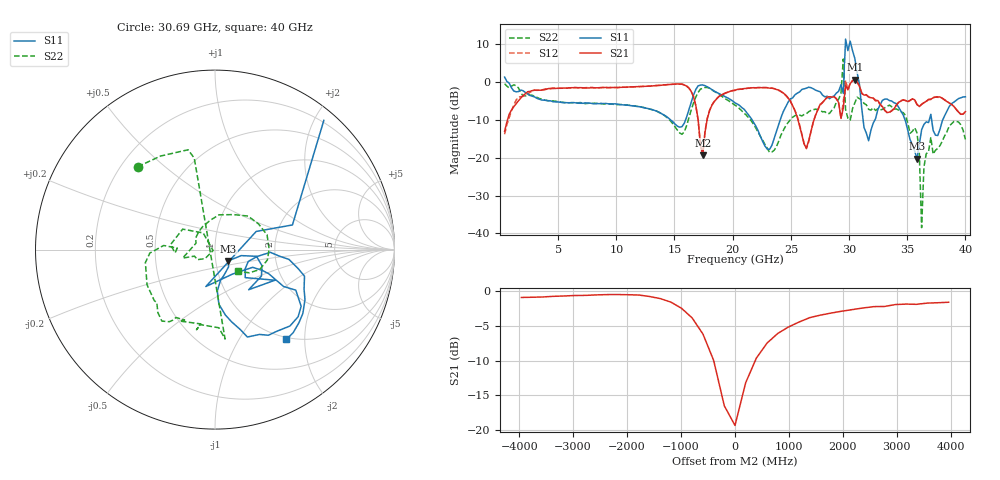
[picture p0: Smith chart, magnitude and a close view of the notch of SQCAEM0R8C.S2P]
! Network Analyzer HP8722ES.07.66: Jul 25, 2000 Serial No. US39175408
! 26 Oct 2004  09:32:31
! Frequency  S11  S21  S12  S22
# HZ  S  DB R  50
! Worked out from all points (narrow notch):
!   201 points, 400 MHz to 40 GHz, reference 50 ohm
!   highest |S21| = 0.61 dB at 30.5 GHz (marker M1); lowest = -19.3 dB at 17.43 GHz (marker M2)
!   notch at M2: 16.8 dB deep, 691 MHz wide at half that depth
!   lowest |S11| = -20.3 dB at 35.84 GHz (marker M3), VSWR 1.21, Z = 57.5 - j7.3 ohm
!   |S11| at or under -10 dB: 14.66 GHz to 15.95 GHz (1.287 GHz wide, 8.41 % of centre); 21.67 GHz to 24.09 GHz (2.415 GHz wide, 10.6 % of centre); 34.81 GHz to 36.9 GHz (2.081 GHz wide, 5.8 % of centre)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
!   |S22| runs from -38.5 to 6.1 dB; largest |S21 - S12| = 0.26
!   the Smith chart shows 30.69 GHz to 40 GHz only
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4e8  1.31 -10.9  -13.01 79.4  -13.79 83.7  -0.44 -5.1
7.132e9  -5.60 -84.4  -1.52 -7.7  -1.53 -8.7  -5.62 -113.3
1.3666e10  -7.94 -83.6  -0.87 -37.5  -0.85 -38.1  -8.04 -172.0
1.6042e10  -9.26 -21.5  -1.07 -73.4  -1.03 -73.5  -11.50 41.4
1.7428e10  -0.76 -52.4  -19.32 -30.6  -19.09 -28.2  -1.64 -77.5
2.02e10  -5.49 -86.0  -2.20 -36.9  -2.09 -37.0  -6.10 -167.8
2.317e10  -17.77 -31.4  -1.61 -69.9  -1.50 -69.9  -18.59 79.6
2.6932e10  -1.77 -49.7  -10.48 -18.8  -10.60 -19.3  -7.28 -110.6
2.8714e10  -3.67 -40.4  -3.88 -54.4  -3.82 -54.6  -6.85 119.2
2.9506e10  -2.97 2.7  -6.87 -170.6  -5.26 -148.7  6.09 28.4
2.9704e10  11.37 -8.3  -0.87 -30.8  0.47 -18.0  -7.29 -55.4
2.9902e10  8.32 -57.7  -2.05 -25.6  -2.02 -25.8  -9.54 4.6
3.01e10  10.84 -76.8  -0.40 -32.3  -0.37 -32.4  -10.08 4.9
3.0496e10  6.27 -107.7  0.61 -58.2  0.71 -58.0  -5.51 -29.4
3.0694e10  2.52 44.6  0.06 -74.4  -0.11 -75.1  -3.99 133.0
3.1288e10  -12.01 23.8  -3.46 -80.5  -3.54 -80.8  -5.64 102.8
3.1486e10  -13.47 -103.9  -3.32 -78.3  -3.42 -78.8  -5.99 -83.6
3.3466e10  -4.88 -53.0  -7.95 -67.8  -8.04 -68.5  -6.08 -126.6
3.5842e10  -20.27 -40.5  -5.90 -77.4  -5.94 -77.7  -13.43 147.6
3.6238e10  -12.61 -9.2  -5.86 -67.2  -5.93 -68.1  -38.48 -152.9
3.703e10  -8.52 -27.0  -4.53 -70.1  -4.62 -70.8  -14.58 -165.3
4e10  -3.89 -51.5  -7.79 -78.4  -7.87 -78.2  -15.17 -43.8
